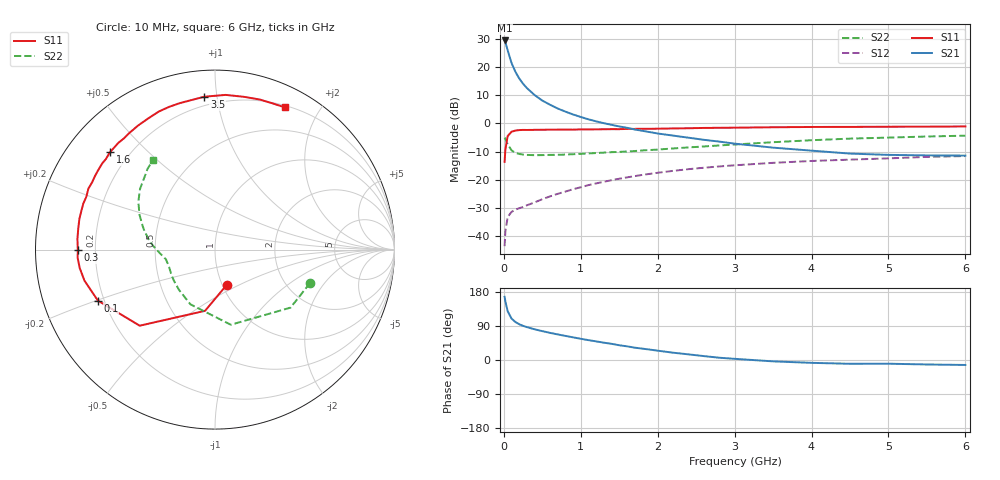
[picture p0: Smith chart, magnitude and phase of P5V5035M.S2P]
! SIEMENS Small Signal Semiconductors
! BFP183
! Si NPN RF Bipolar Junction Transistor in SOT143
! VCE = 0.5 V  IC = 35 mA
! Common Emitter S-Parameters:  March  1996
# GHz  S  MA  R  50
!  f  S11  S21  S12  S22
! GHz  MAG  ANG  MAG  ANG  MAG  ANG  MAG  ANG
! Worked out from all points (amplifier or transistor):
!   36 points, 10 MHz to 6 GHz, reference 50 ohm
!   highest |S21| = 29.4 dB at 10 MHz (marker M1)
!   |S21| within 3 dB of that: start of sweep to 44.65 MHz
!   unconditionally stable (mu >= 1): start of sweep to 18.38 MHz; 183.4 MHz to end of sweep
!   at 250 MHz: K = 1.23, MAG = 18.9 dB, |S12| = -29.6 dB
!   at 1.4 GHz: K = 2.01, MAG = 4.0 dB, |S12| = -20.1 dB
!   at 6 GHz: K = 1.52, MAG = -4.2 dB, |S12| = -11.6 dB
!   S11 on the Smith chart (normalised r, x): 10 MHz: 1.05, -0.43; 100 MHz: 0.18, -0.20; 300 MHz: 0.13, -0.00; 1.6 GHz: 0.13, +0.39; 3.5 GHz: 0.15, +0.92; 6 GHz: 0.22, +1.58
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0.01  0.2081 -72.0  29.39 166.6  0.0067 69.4  0.5611 -19.4
0.02  0.3456 -99.2  27.41 154.5  0.0124 62.5  0.5309 -37.5
0.05  0.5964 -134.7  19.6 128.7  0.022 46.6  0.4278 -78.1
0.1  0.7117 -156.5  11.73 109.4  0.0271 34.2  0.3344 -114.1
0.15  0.7474 -166.6  8.216 100.3  0.0297 33.3  0.3006 -132.1
0.2  0.7606 -172.2  6.238 94.4  0.0315 34.9  0.2872 -142.6
0.25  0.7667 -176.6  5.027 90.1  0.0331 36.3  0.2808 -149.4
0.3  0.7644 -179.7  4.217 86.8  0.0355 39.0  0.2765 -154.0
0.4  0.7688 175.5  3.174 81.0  0.0399 43.6  0.2734 -159.9
0.5  0.7709 171.1  2.536 76.2  0.0455 46.3  0.2745 -163.5
0.6  0.7747 167.2  2.14 71.6  0.051 49.2  0.2768 -166.2
0.7  0.7752 163.9  1.834 67.5  0.0566 50.7  0.2778 -168.1
0.8  0.7773 160.7  1.616 63.6  0.062 52.0  0.2805 -169.4
1.1  0.7806 151.3  1.18 52.4  0.0807 52.6  0.2938 -173.2
1.3  0.787 145.8  1.008 45.7  0.0926 51.7  0.3037 -175.3
1.6  0.7978 137.2  0.836 36.1  0.1105 49.4  0.318 -178.4
2.2  0.8133 121.8  0.608 19.3  0.1444 42.8  0.3598 173.8
2.8  0.8354 107.8  0.476 6.0  0.1729 35.2  0.4069 165.2
3.5  0.8539 94.0  0.372 -3.6  0.2002 26.8  0.4642 155.1
4.5  0.8666 79.1  0.292 -10.0  0.2282 15.3  0.5375 141.0
5.5  0.8754 68.6  0.271 -11.8  0.2551 5.7  0.5857 130.0
6  0.8827 63.9  0.269 -13.1  0.264 0.6  0.606 124.9
